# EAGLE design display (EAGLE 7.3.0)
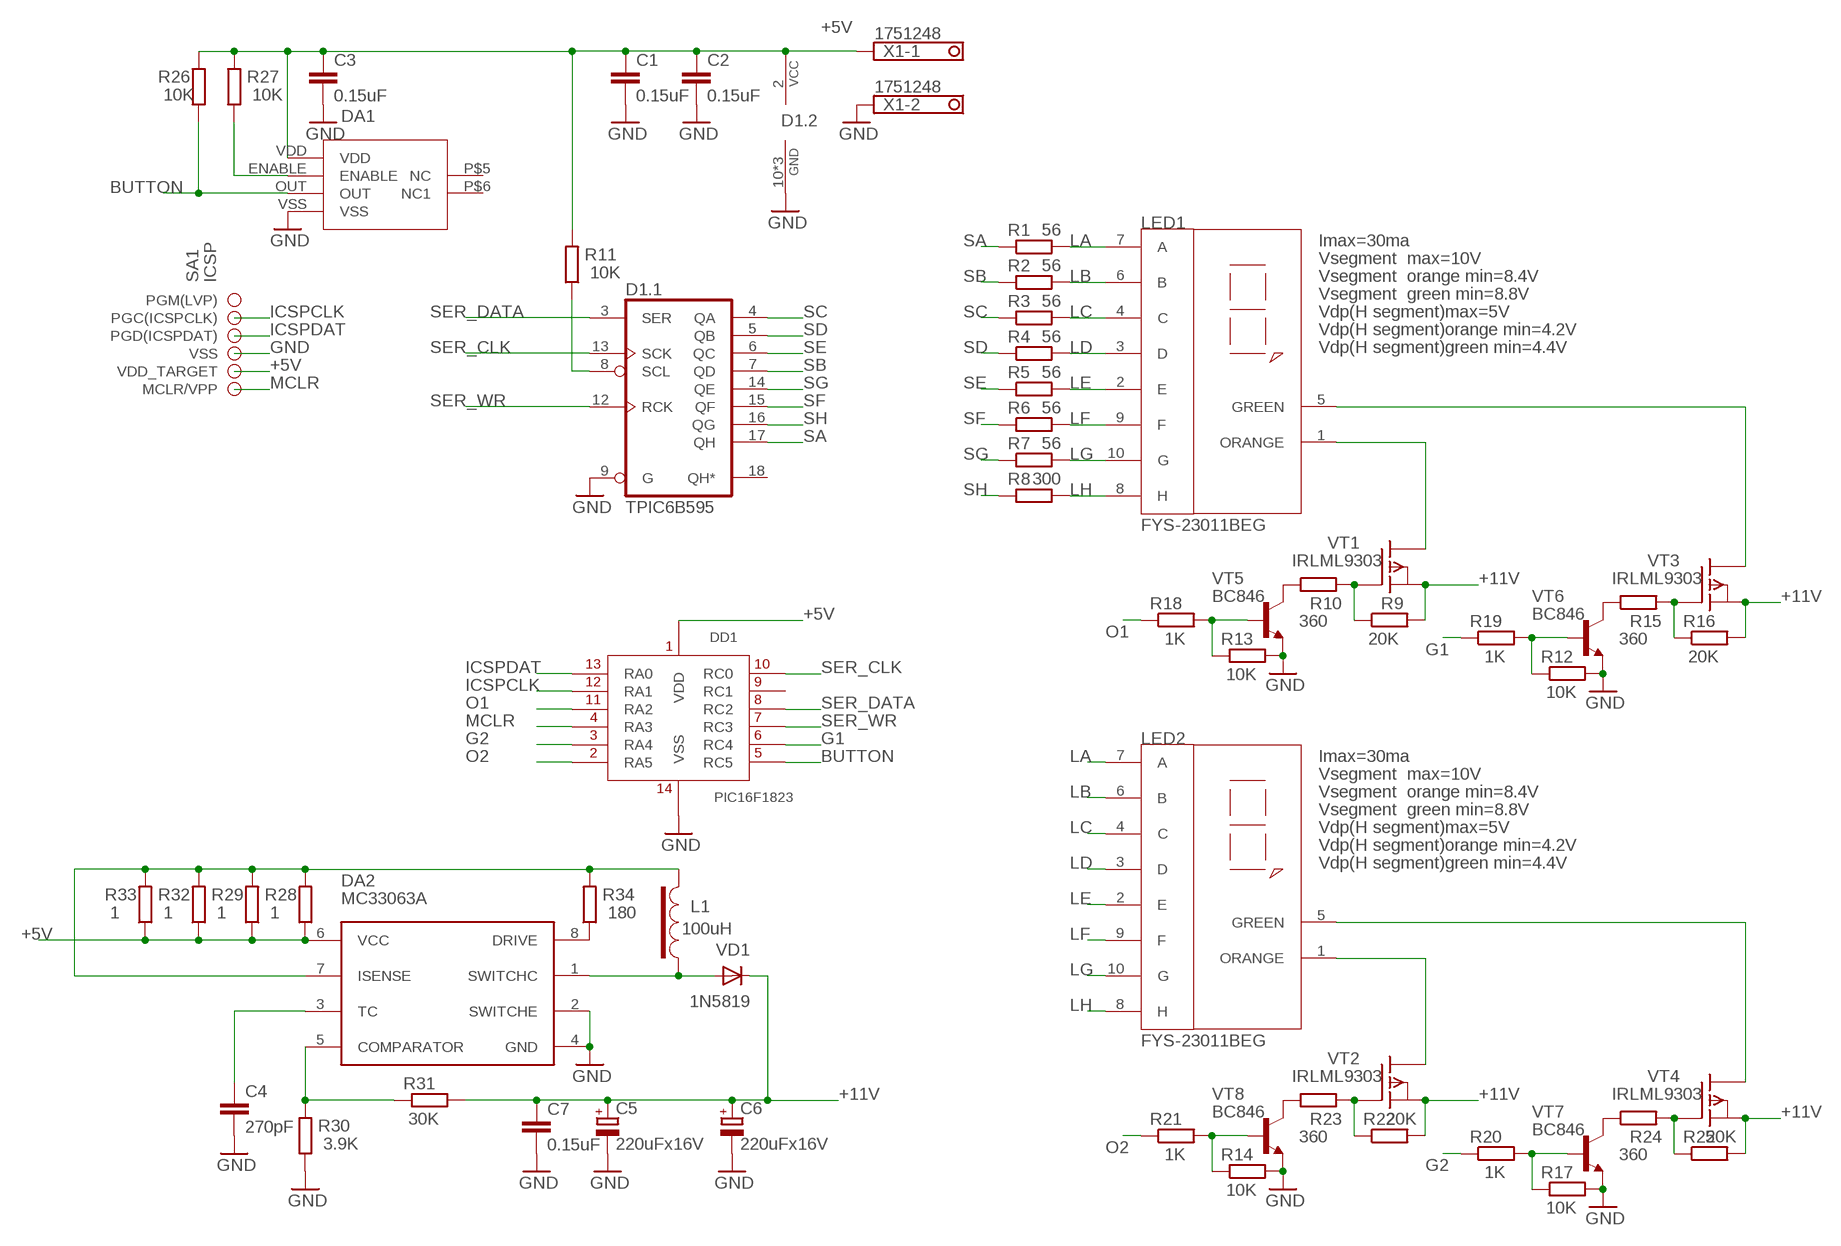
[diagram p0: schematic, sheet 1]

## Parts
C1  0.15uF  C-EUC0805  [C0805]
C2  0.15uF  C-EUC0805  [C0805]
C3  0.15uF  C-EUC0805  [C0805]
C4  270pF  C-EUC0805  [C0805]
C5  220uFx16V  CPOL-EU175TMP-0810  [175TMP-0810]
C6  220uFx16V  CPOL-EU175TMP-0810  [175TMP-0810]
C7  0.15uF  C-EUC0805  [C0805]
D1  TPIC6B595  TPIC6B595SOIC20  [SO20L]
DA1  HALL_BUTTON  [HALL_BUTTON]
DA2  MC33063A  MC34063ASOIC8  [SOIC8]
DD1  PIC16F1823  PIC16F1823SOIC14  [SO14]
L1  100uH  INDUCTOR  [0914]
LED1  FYS-23011BEG  FYS-23011  [FYS-23011]
LED2  FYS-23011BEG  FYS-23011  [FYS-23011]
R1  56  R-EU_R0805  [R0805]
R2  56  R-EU_R0805  [R0805]
R3  56  R-EU_R0805  [R0805]
R4  56  R-EU_R0805  [R0805]
R5  56  R-EU_R0805  [R0805]
R6  56  R-EU_R0805  [R0805]
R7  56  R-EU_R0805  [R0805]
R8  300  R-EU_R0805  [R0805]
R9  20K  R-EU_R0805  [R0805]
R10  360  R-EU_R0805  [R0805]
R11  10K  R-EU_R0805  [R0805]
R12  10K  R-EU_R0805  [R0805]
R13  10K  R-EU_R0805  [R0805]
R14  10K  R-EU_R0805  [R0805]
R15  360  R-EU_R0805  [R0805]
R16  20K  R-EU_R0805  [R0805]
R17  10K  R-EU_R0805  [R0805]
R18  1K  R-EU_R0805  [R0805]
R19  1K  R-EU_R0805  [R0805]
R20  1K  R-EU_R0805  [R0805]
R21  1K  R-EU_R0805  [R0805]
R22  20K  R-EU_R0805  [R0805]
R23  360  R-EU_R0805  [R0805]
R24  360  R-EU_R0805  [R0805]
R25  20K  R-EU_R0805  [R0805]
R26  10K  R-EU_R0805  [R0805]
R27  10K  R-EU_R0805  [R0805]
R28  1  R-EU_R0805  [R0805]
R29  1  R-EU_R0805  [R0805]
R30  3.9K  R-EU_R0805  [R0805]
R31  30K  R-EU_R0805  [R0805]
R32  1  R-EU_R0805  [R0805]
R33  1  R-EU_R0805  [R0805]
R34  180  R-EU_R0805  [R0805]
SA1  ICSP  [ICSP]
VD1  1N5819  SM5819  [MELF-MLL41]
VT1  IRLML9303  P-MOSFETSOT23  [SOT23]
VT2  IRLML9303  P-MOSFETSOT23  [SOT23]
VT3  IRLML9303  P-MOSFETSOT23  [SOT23]
VT4  IRLML9303  P-MOSFETSOT23  [SOT23]
VT5  BC846  BC846-NPN-SOT23-BEC  [SOT23-BEC]
VT6  BC846  BC846-NPN-SOT23-BEC  [SOT23-BEC]
VT7  BC846  BC846-NPN-SOT23-BEC  [SOT23-BEC]
VT8  BC846  BC846-NPN-SOT23-BEC  [SOT23-BEC]
X1  1751248  [1751248]

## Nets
+5V: C1.1 C2.1 C3.1 D1.2(.2:VCC) DA1.VDD DA2.6(VCC) DD1.1(VDD) R11.2 R26.2 R27.2 R28.1 R29.1 R32.1 R33.1 SA1.VDD(VDD_TARGET) X1.1
+11V: C5.+ C6.+ C7.1 R9.2 R16.2 R22.2 R25.2 R31.2 VD1.C VT1.2(S) VT2.2(S) VT3.2(S) VT4.2(S)
BUTTON: DA1.OUT DD1.5(RC5) R26.1
G1: DD1.6(RC4) R19.1
G2: DD1.3(RA4) R20.1
GND: C1.2 C2.2 C3.2 C4.2 C5.- C6.- C7.2 D1.9(.1:G) D1.10(.2:GND) D1.11(.2:GND) D1.19(.2:GND) DA1.VSS DA2.2(SWITCHE) DA2.4(GND) DD1.14(VSS) R12.2 R13.2 R14.2 R17.2 R30.1 SA1.VSS VT5.E VT6.E VT7.E VT8.E X1.2
ICSPCLK: DD1.12(RA1) SA1.PGC(ICSPCLK)
ICSPDAT: DD1.13(RA0) SA1.PGD(ICSPDAT)
LA: LED1.7(A) LED2.7(A) R1.2
LB: LED1.6(B) LED2.6(B) R2.2
LC: LED1.4(C) LED2.4(C) R3.2
LD: LED1.3(D) LED2.3(D) R4.2
LE: LED1.2(E) LED2.2(E) R5.2
LF: LED1.9(F) LED2.9(F) R6.2
LG: LED1.10(G) LED2.10(G) R7.2
LH: LED1.8(H) LED2.8(H) R8.2
MCLR: DD1.4(RA3) SA1.MCLR/VPP
N$1: R10.1 VT5.C
N$2: D1.8(.1:SCL) R11.1
N$3: R15.1 VT6.C
N$4: R24.1 VT7.C
N$5: R23.1 VT8.C
N$6: R13.1 R18.2 VT5.B
N$7: R12.1 R19.2 VT6.B
N$8: R17.1 R20.2 VT7.B
N$9: LED1.1(ORANGE) VT1.3(D)
N$10: R9.1 R10.2 VT1.1(G)
N$11: R14.1 R21.2 VT8.B
N$12: C4.1 DA2.3(TC)
N$13: DA1.ENABLE R27.1
N$14: DA2.5(COMPARATOR) R30.2 R31.1
N$15: R15.2 R16.1 VT3.1(G)
N$16: LED1.5(GREEN) VT3.3(D)
N$17: DA2.7(ISENSE) L1.L2 R28.2 R29.2 R32.2 R33.2 R34.2
N$18: DA2.1(SWITCHC) L1.L1 VD1.A
N$24: DA2.8(DRIVE) R34.1
N$37: LED2.1(ORANGE) VT2.3(D)
N$38: R22.1 R23.2 VT2.1(G)
N$39: R24.2 R25.1 VT4.1(G)
N$40: LED2.5(GREEN) VT4.3(D)
O1: DD1.11(RA2) R18.1
O2: DD1.2(RA5) R21.1
SA: D1.17(.1:QH) R1.1
SB: D1.7(.1:QD) R2.1
SC: D1.4(.1:QA) R3.1
SD: D1.5(.1:QB) R4.1
SE: D1.6(.1:QC) R5.1
SER_CLK: D1.13(.1:SCK) DD1.10(RC0)
SER_DATA: D1.3(.1:SER) DD1.8(RC2)
SER_WR: D1.12(.1:RCK) DD1.7(RC3)
SF: D1.15(.1:QF) R6.1
SG: D1.14(.1:QE) R7.1
SH: D1.16(.1:QG) R8.1
Unconnected: D1.18(.1:QH*) DA1.P$5(NC) DA1.P$6(NC1) DD1.9(RC1) SA1.PGM(LVP)

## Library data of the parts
C1-C4 C7 = resistors:C-EU: CAPACITOR, European symbol
C5 C6 = resistors:CPOL-EU: POLARIZED CAPACITOR, European symbol
D1 = 74xx:TPIC6B595
DA1 = button:HALL_BUTTON
DA2 = power:MC34063A
DD1 = Microchip:PIC16F1823
L1 = inductors:INDUCTOR
LED1 LED2 = led:FYS-23011
R1-R34 = resistors:R-EU_: RESISTOR, European symbol
SA1 = connectors:ICSP
VD1 = diodes:SM5819
VT1-VT4 = Tranzistors:P-MOSFET
VT5-VT8 = Tranzistors:*-NPN-: NPN Transistror BF959 corrected 2008.03.06
X1 = connectors:1751248: MKDS 1/ 2-3,5 Printklemme; OC_FARNELL: unknown; OC_NEWARK: unknown

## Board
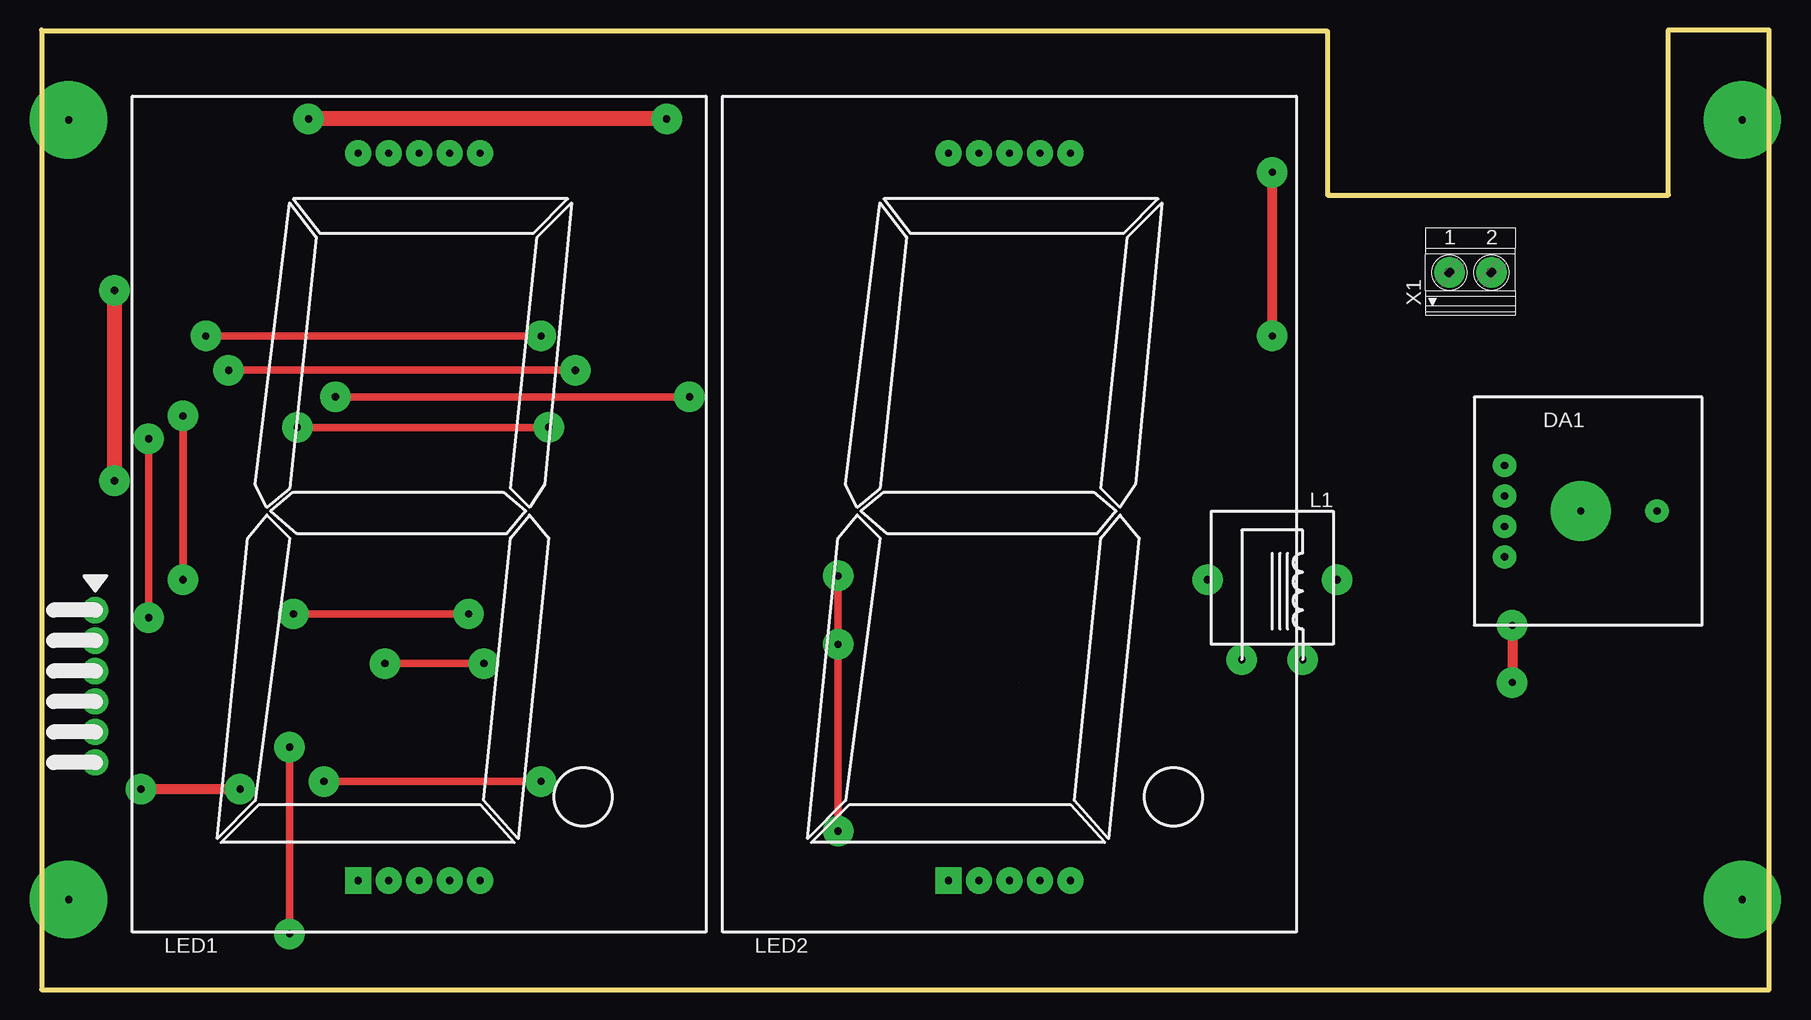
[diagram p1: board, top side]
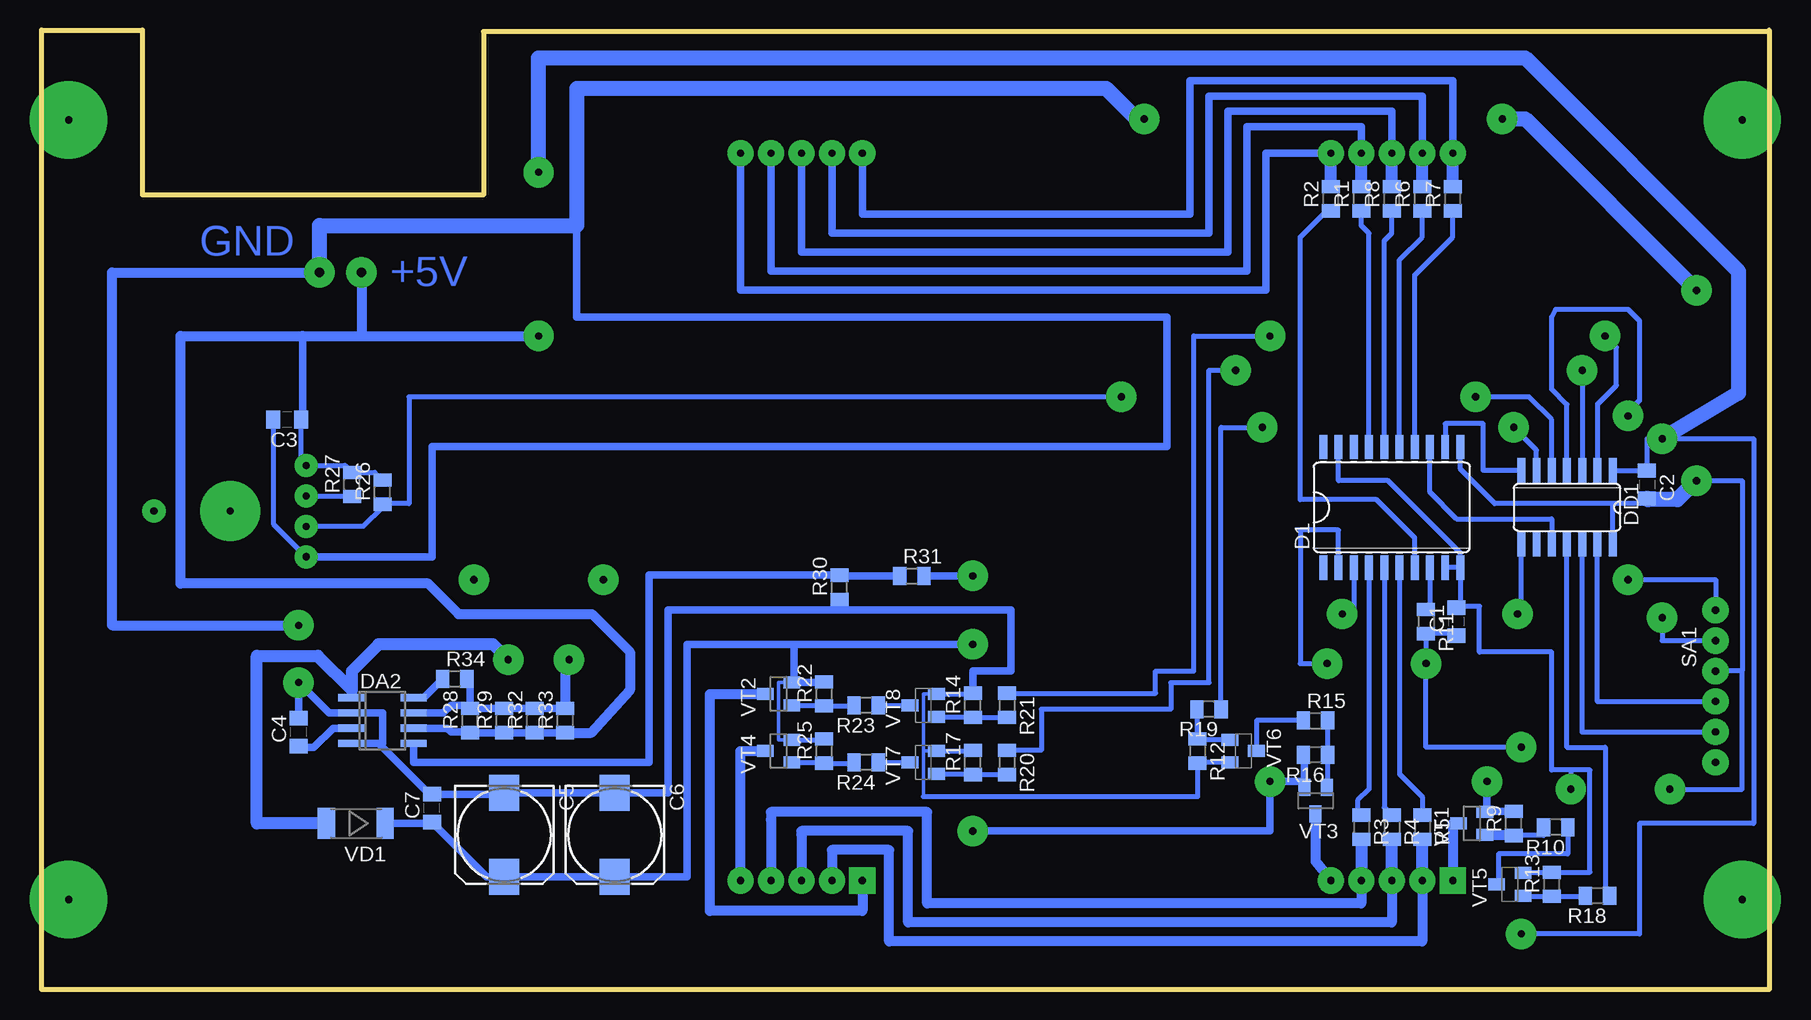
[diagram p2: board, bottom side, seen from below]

Size 144 x 80 mm. Coordinates in mm from the lower left corner, seen from the top.
Outline: 0,80 0,0 144,0 144,80 135.6,80 135.6,66.24 107.18,66.24 107.18,79.89 0.03,79.89
Copper layers (1*16): Top 0.035mm / dielectric 1.5mm / Bottom 0.035mm
Design rules "default": minimum track width 10mil, minimum drill 24mil, track to track 8mil, track to pad 8mil, pad to pad 8mil, via to via 8mil, smd to smd 8mil, copper to edge 40mil, drill to drill 8mil, minimum pad ring 10mil, minimum via ring 8mil, stop-mask expansion 4mil, vias tented up to drill 0mil, thermal gap 10mil

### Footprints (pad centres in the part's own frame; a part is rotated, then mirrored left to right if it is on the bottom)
C0805 = smd 1.2 x 1.5: 1 -1.167,0; 2 1.167,0
175TMP-0810 = smd 3 x 2.5: + 3.5,0; - -3.5,0
SO20L = smd 0.66 x 2.032: 1 -5.715,-5.029; 2 -4.445,-5.029; 3 -3.175,-5.029; 4 -1.905,-5.029; 5 -0.635,-5.029; 6 0.635,-5.029; 7 1.905,-5.029; 8 3.175,-5.029; 9 4.445,-5.029; 10 5.715,-5.029; 11 5.715,5.029; 12 4.445,5.029; 13 3.175,5.029; 14 1.905,5.029; 15 0.635,5.029; 16 -0.635,5.029; 17 -1.905,5.029; 18 -3.175,5.029; 19 -4.445,5.029; 20 -5.715,5.029
HALL_BUTTON = drill 0.6 pad 1.93: ENABLE 0,-2.54; OUT 0,-5.08; P$5 12.7,-3.81; VDD 0,0; VSS 0,-7.62 | drill 0.6 pad 5: P$6 6.35,-3.81
SOIC8 = smd 0.6 x 2.2: 1 -1.905,-2.6; 2 -0.635,-2.6; 3 0.635,-2.6; 4 1.905,-2.6; 5 1.905,2.6; 6 0.635,2.6; 7 -0.635,2.6; 8 -1.905,2.6
SO14 = smd 0.66 x 2.032: 1 -3.81,-3.073; 2 -2.54,-3.073; 3 -1.27,-3.073; 4 0,-3.073; 5 1.27,-3.073; 6 2.54,-3.073; 7 3.81,-3.073; 8 3.81,3.073; 9 2.54,3.073; 10 1.27,3.073; 11 0,3.073; 12 -1.27,3.073; 13 -2.54,3.073; 14 -3.81,3.073
0914 = drill 0.6 pad 2.54: L1 0,0; L2 5.08,0; NC1 -2.857,-6.668; NC2 7.938,-6.668
FYS-23011 = drill 0.6 pad 2.184 square: 1 0,-60.642 | drill 0.6 pad 2.184: 2 2.54,-60.642; 3 5.08,-60.642; 4 7.62,-60.642; 5 10.16,-60.642; 6 10.16,0; 7 7.62,0; 8 5.08,0; 9 2.54,0; 10 0,0
R0805 = smd 1.1 x 1.5: 1 -1.009,0; 2 1.009,0
ICSP = drill 0.6 pad 2.184: MCLR/VPP 0,0; PGC(ICSPCLK) 10.16,0; PGD(ICSPDAT) 7.62,0; PGM(LVP) 12.7,0; VDD 2.54,0; VSS 5.08,0
MELF-MLL41 = smd 1.45 x 2.6: A 2.445,0; C -2.445,0
SOT23 = smd 1 x 1.4: 1 -0.95,-1.1; 2 0.95,-1.1; 3 0,1.1
SOT23-BEC = smd 1 x 1.4: B -0.95,-1.1; C 0,1.1; E 0.95,-1.1
1751248 = drill 0.8 pad 2.54: 1 -1.75,-0.1; 2 1.75,-0.1

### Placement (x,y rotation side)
C1  26.06,30.68 90 bottom
C2  10.19,42.11 270 bottom
C3  123.53,47.51 180 bottom
C4  122.58,21.47 90 bottom
C5  105.44,12.9 270 bottom
C6  96.23,12.9 270 bottom
C7  111.47,15.12 90 bottom
D1  31.46,40.2 0 bottom
DA1  121.95,43.7 0 top
DA2  115.6,22.42 270 bottom
DD1  16.86,40.2 180 bottom
L1  105.12,27.5 180 top
LED1  26.38,69.73 0 top
LED2  75.59,69.73 0 top
R1  34,65.92 90 bottom
R2  36.54,65.92 90 bottom
R3  34,13.53 270 bottom
R4  31.46,13.53 270 bottom
R5  28.92,13.53 270 bottom
R6  28.92,65.92 90 bottom
R7  26.38,65.92 90 bottom
R8  31.46,65.92 90 bottom
R9  21.3,13.85 90 bottom
R10  17.81,13.53 180 bottom
R11  28.6,30.68 270 bottom
R12  47.65,19.88 270 bottom
R13  18.12,8.77 90 bottom
R14  66.39,23.69 90 bottom
R15  37.81,22.42 0 bottom
R16  37.81,19.56 180 bottom
R17  66.39,18.93 90 bottom
R18  14.31,7.82 180 bottom
R19  46.7,23.38 180 bottom
R20  63.53,18.93 270 bottom
R21  63.53,23.69 270 bottom
R22  78.77,24.64 90 bottom
R23  75.28,23.69 180 bottom
R24  75.28,18.93 180 bottom
R25  78.77,19.88 90 bottom
R26  115.6,41.47 90 bottom
R27  118.14,42.11 90 bottom
R28  108.3,22.42 90 bottom
R29  105.44,22.42 90 bottom
R30  77.5,33.53 90 bottom
R31  71.47,34.49 0 bottom
R32  102.9,22.42 90 bottom
R33  100.36,22.42 90 bottom
R34  109.56,25.91 0 bottom
SA1  4.47,31.63 270 top
VD1  117.82,13.85 180 bottom
VT1  24.79,13.85 90 bottom
VT2  82.58,24.64 90 bottom
VT3  37.81,15.76 180 bottom
VT4  82.58,19.88 90 bottom
VT5  21.62,8.77 90 bottom
VT6  43.84,19.88 270 bottom
VT7  70.51,18.93 90 bottom
VT8  70.51,23.69 90 bottom
X1  119.09,59.89 0 top

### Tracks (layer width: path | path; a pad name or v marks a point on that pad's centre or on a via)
+5V  (via drill 0.6 pad 2.54)
  Top 0.61: v28.6,27.18 v36.86,27.18 | v8.92,31 v8.92,45.92 | v20.66,4.64 v20.66,20.2
  Top 0.813: v102.58,54.49 v102.58,68.14
  Bottom 0.406: DD1.1 C2.1 10.19,45.92 v8.92,45.92 1.3,45.92 1.3,13.85 10.82,13.85 10.82,4.64 v20.66,4.64 | C1.1 26.06,29.67 R11.2 v28.6,27.18 28.6,20.2 v20.66,20.2 | R26.2 116.23,43.12 R27.2 118.72,43.7 DA1.VDD 122.37,43.7 C3.1 | D1.2 35.91,38.3 39.08,38.3 39.08,27.18 v36.86,27.18 | v8.92,31 8.92,29.09 SA1.VDD
  Bottom 0.61: DA2.6 110.2,21.79 109.88,21.47 108.35,21.47 R28.1 R29.1 R32.1 R33.1 | C3.1 122.27,47.51 122.27,54.49
  Bottom 0.813: R33.1 98.19,21.41 94.96,24.96 94.96,28.14 98.14,31.31 109.25,31.31 111.79,33.85 132.43,33.85 132.43,54.49 122.27,54.49 117.34,54.49 | 117.34,54.49 v102.58,54.49 | X1.1 117.34,54.49
  Bottom 1.016: 2.57,59.89 2.57,59.57
  Bottom 1.27: 2.57,59.57 2.57,49.73 v8.92,45.92 | 2.57,59.89 20.35,77.67 102.58,77.67 v102.58,68.14
+11V  (via drill 0.6 pad 2.54)  (1 unrouted)
  Top 0.61: v23.52,17.34 v41.62,17.34 | v66.39,13.21 v66.39,28.77 v66.39,34.49
  Bottom 0.305: VT4.2 82.58,20.83 82.58,25.6 VT2.2
  Bottom 0.406: VT4.2 78.77,20.83 R25.2
  Bottom 0.61: R9.2 23.69,14.86 VT1.2 23.52,14.8 v23.52,17.34 | R16.2 38.76,19.56 VT3.2 38.76,17.34 v41.62,17.34 41.62,13.21 v66.39,13.21 | v66.39,28.77 81.31,28.77 | 81.31,28.77 90.2,28.77 90.2,9.4 C6.+ C5.+ 106.92,9.4 C7.1 111.57,13.85 VD1.C | VT2.2 78.82,25.6 R22.2 | R31.2 v66.39,34.49 | VT2.2 81.31,25.59 81.31,28.77
BUTTON  (via drill 0.6 pad 2.54)
  Top 0.61: v24.48,49.41 v54,49.41
  Bottom 0.406: R26.1 115.6,40.2 117.19,38.61 DA1.OUT | DD1.5 18.12,47.51 20.03,49.41 v24.48,49.41 | 115.34,40.2 R26.1 | v54,49.41 113.38,49.41 113.38,40.52 115.6,40.52 R26.1
G1  (via drill 0.6 pad 2.54)
  Top 0.61: v42.26,46.87 v21.3,46.87
  Bottom 0.406: R19.1 45.69,46.87 v42.26,46.87 | DD1.6 19.39,44.97 v21.3,46.87
G2  (via drill 0.6 pad 2.54)
  Top 0.61: v44.48,51.63 v15.59,51.63
  Bottom 0.406: v44.48,51.63 46.7,51.63 46.7,25.6 49.88,25.6 49.88,23.38 60.67,23.38 60.67,19.94 R20.1 | v15.59,51.63 DD1.3
GND  (via drill 0.6 pad 2.54)
  Top 0.813: v16.54,16.71 v8.28,16.71 | v122.58,30.36 v122.58,25.6
  Top 1.27: v52.1,72.59 v22.25,72.59 | v6.06,58.3 v6.06,42.42
  Bottom 0.305: VT7.E 70.51,19.88 | 70.51,19.88 70.51,24.64 VT8.E | 70.51,16.07 70.51,19.88
  Bottom 0.406: VT7.E 66.39,19.88 R17.2 | VT8.E 66.39,24.64 R14.2 | VT6.E 47.65,18.93 R12.2 47.65,16.07 70.51,16.07 | VT5.E 20.52,9.78 R13.2 14.95,9.78 14.95,18.3 16.54,18.3 | DD1.14 13.04,40.52 | 13.04,40.52 22.89,40.52 25.75,43.38 D1.11 | 13.04,40.52 10.19,40.52 C2.2 10.19,40.84 | D1.10 D1.9 | D1.10 25.75,31.84 C1.2 26.06,31.95 24.16,31.95 24.16,28.14 18.12,28.14 18.12,18.3 16.54,18.3 | C3.2 124.7,38.83 DA1.VSS | 16.54,18.3 v16.54,16.71 | 6.7,41.79 v6.06,42.42 2.25,42.42 2.25,26.55 | D1.19 35.91,42.42 31.78,42.42 25.75,36.39 D1.10 | 2.25,26.55 SA1.VSS | v8.28,16.71 2.25,16.71 2.25,26.55
  Bottom 0.61: R14.2 66.39,26.55 63.21,26.55 63.21,31.63 77.5,31.63 | 77.5,31.63 91.78,31.63 91.78,16.4 C6.- C5.- 105.55,16.29 C7.2 111.57,16.39 111.79,16.39 115.92,20.52 | R30.1 77.5,31.63 | DA2.4 115.92,20.52 | 115.92,20.52 115.6,20.52 115.6,23.06 DA2.2 120.04,23.06 v122.58,25.6 C4.2 | DA1.VSS 111.47,36.08 111.47,45.28 50.19,45.28 50.19,56.08 99.41,56.08 99.41,64.02
  Bottom 0.813: v122.58,30.36 138.14,30.36 138.14,59.79 X1.2
  Bottom 1.27: v22.25,72.59 20.35,72.59 v6.06,58.3 | v6.06,42.42 7.65,40.84 10.09,40.84 C2.2 | v52.1,72.59 52.73,72.59 55.27,75.13 99.41,75.13 99.41,64.02 99.41,63.7 120.84,63.7 X1.2
ICSPCLK
  Bottom 0.406: DD1.12 15.59,21.47 SA1.PGC(ICSPCLK)
ICSPDAT
  Bottom 0.406: DD1.13 14.31,24.01 SA1.PGD(ICSPDAT)
LA
  Bottom 0.61: LED1.7 34,71.95 43.52,71.95 43.52,59.89 83.21,59.89 LED2.7
  Bottom 1.016: R1.2 LED1.7
LB
  Bottom 0.61: LED1.6 41.94,69.73 41.94,58.3 85.75,58.3 LED2.6
  Bottom 1.016: R2.2 LED1.6
LC
  Bottom 0.813: LED1.4 34,7.18 70.19,7.18 70.19,14.8 83.21,14.8 83.21,14.17 LED2.4
  Bottom 1.016: R3.2 LED1.4
LD
  Bottom 0.813: LED1.3 31.46,5.59 71.78,5.59 71.78,13.21 80.67,13.21 80.67,12.9 LED2.3
  Bottom 1.016: LED1.3 R4.2
LE
  Bottom 0.813: LED1.2 28.92,4.01 73.37,4.01 73.37,11.63 78.13,11.63 LED2.2
  Bottom 1.016: LED1.2 R5.2
LF
  Bottom 0.61: LED1.9 28.92,74.49 46.7,74.49 46.7,63.06 78.13,63.06 LED2.9
  Bottom 1.016: R6.2 LED1.9
LG
  Bottom 0.61: LED1.10 26.38,75.76 48.29,75.76 48.29,64.65 75.59,64.65 LED2.10
  Bottom 1.016: R7.2 LED1.10
LH
  Bottom 0.61: LED1.8 31.46,73.22 45.11,73.22 45.11,61.48 80.67,61.48 LED2.8
  Bottom 1.016: R8.2 LED1.8
MCLR  (via drill 0.6 pad 2.54)
  Top 0.61: v11.78,47.82 v11.78,34.17
  Bottom 0.406: DD1.4 16.86,48.77 18.12,50.05 18.12,56.08 17.81,56.71 11.78,56.71 10.82,55.76 10.82,49.09 11.78,48.14 v11.78,47.82 | v11.78,34.17 4.47,34.17 SA1.MCLR/VPP
N$1
  Bottom 0.406: R10.1 16.8,11.31 22.57,11.31 22.57,9.09 VT5.C
N$2
  Bottom 0.406: D1.8 28.29,31.69 R11.1
N$3
  Bottom 0.406: R15.1 42.74,22.42 VT6.C
N$4
  Bottom 0.406: R24.1 VT7.C
N$5
  Bottom 0.406: R23.1 VT8.C
N$6
  Bottom 0.406: VT5.B 20.52,7.76 R13.1 15.32,7.76 R18.2
N$7
  Bottom 0.406: VT6.B 47.65,20.83 R12.1 47.65,23.32 R19.2
N$8
  Bottom 0.406: VT7.B 66.39,17.98 R17.1 R20.2
N$9
  Bottom 0.813: VT1.3 26.38,13.85 LED1.1
N$10
  Bottom 0.406: R10.2 18.82,12.84 R9.1
  Bottom 0.813: VT1.1 21.3,12.9 R9.1
N$11
  Bottom 0.406: VT8.B 66.39,22.74 R14.1 R21.2
N$12
  Bottom 0.61: DA2.3 119.72,21.79 121.31,20.2 122.48,20.2 C4.1
N$13
  Bottom 0.406: R27.1 121.89,41.1 DA1.ENABLE
N$14
  Bottom 0.61: R31.1 77.5,34.49 R30.2 93.37,34.54 93.37,18.93 113,18.93 DA2.5
N$15
  Bottom 0.406: VT3.1 37.12,17.11 36.8,17.11 R16.1 R15.2
N$16
  Bottom 0.813: VT3.3 37.81,10.68 LED1.5
N$17
  Bottom 0.61: DA2.7 110.52,23.06 109.88,23.69 108.56,23.69 R28.2 | R28.2 R29.2 R32.2 R33.2 | R28.2 108.3,25.65 R34.2
  Bottom 0.813: L1.L2 100.36,27.5 R33.2
N$18
  Bottom 0.61: 118.45,24.33 DA2.1 118.2,24.9 118.14,24.96
  Bottom 1.016: VD1.A 126.08,13.85 126.08,27.82 121,27.82 118.14,24.96 118.14,26.55 115.92,28.77 106.39,28.77 L1.L1
N$19  (via drill 0.6 pad 6.45)
  other vias: 2.25,7.5
N$20  (via drill 0.6 pad 6.45)
  other vias: 141.75,7.5
N$21  (via drill 0.6 pad 6.45)
  other vias: 141.75,72.5
N$22  (via drill 0.6 pad 6.45)
  other vias: 2.25,72.5
N$24
  Bottom 0.61: DA2.8 112.16,24.33 R34.1
N$37
  Bottom 0.813: LED2.1 75.59,6.55 88.29,6.55 88.29,24.64 VT2.3
N$38
  Bottom 0.406: VT2.1 78.77,23.7 R22.1 76.28,23.64 R23.2
N$39
  Bottom 0.406: VT4.1 78.77,18.93 R25.1 76.28,18.87 R24.2
N$40
  Bottom 0.813: LED2.5 85.75,19.88 VT4.3
O1
  Bottom 0.406: DD1.11 16.86,20.2 13.68,20.2 13.68,8.19 R18.1
O2  (via drill 0.6 pad 2.54)
  Top 0.61: v41.62,54.49 v13.68,54.49
  Bottom 0.406: R21.1 51.15,24.7 51.15,26.55 47.97,26.55 47.97,54.49 v41.62,54.49 | DD1.2 14.31,48.77 12.73,50.36 12.73,53.54 v13.68,54.49
SA
  Bottom 0.406: D1.17 33.36,63.06 34,63.7 R1.1
SB
  Bottom 0.406: R2.1 36.91,64.91 39.08,62.74 39.08,40.84 32.73,40.84 29.55,37.66 D1.7
SC
  Bottom 0.406: D1.4 33.36,16.71 34.32,15.76 34.32,14.86 R3.1
SD
  Bottom 0.406: D1.5 32.09,15.18 R4.1
SE
  Bottom 0.406: D1.6 30.82,17.98 28.92,16.07 R5.1
SER_CLK
  Bottom 0.406: DD1.10 18.12,39.25 26.06,39.25 28.29,41.47 D1.13
SER_DATA  (via drill 0.6 pad 2.54)
  Top 0.61: v35.59,31.31 v20.98,31.31
  Bottom 0.406: D1.3 34.63,31.31 v35.59,31.31 | v20.98,31.31 20.66,31.31 DD1.8
SER_WR
  Bottom 0.406: DD1.7 23.84,43.28 23.84,47.19 27.02,47.19 D1.12
SF
  Bottom 0.406: D1.15 30.82,60.84 28.92,62.74 R6.1
SG
  Bottom 0.406: D1.14 29.55,59.57 26.38,62.74 R7.1
SH
  Bottom 0.406: D1.16 32.09,62.43 31.46,63.06 R8.1

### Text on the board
Bottom: GND | +5V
